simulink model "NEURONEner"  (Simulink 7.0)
settings: Solver=ode45  StartTime=0.0  StopTime=tstop  RelTol=1e-3
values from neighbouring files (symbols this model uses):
  beta = 1    [ResCourV1.m]    (also in ResCrV1.m; ResEnerV1.m; Constantes.m = 0.95; ConstantesBck.m = 0.95)
  Cdl = 731.3E-9    (= 7.313e-07)    [ResCourV1.m]    (also in ResCrV1.m; ResEnerV1.m; Constantes.m = 6.03e-07; ConstantesBck.m = 6.03e-07)
  I0Stim = ResSinhCorr(iRes,2)*1E-3    [ResCrV1.m]    (also in ResEnerV1.m; WaveCompIET.m = 0; WaveCompIETIf.m = 0)
  Rct = 605.2E3    (= 605200)    [ResCourV1.m]    (also in ResCrV1.m; ResEnerV1.m; Constantes.m = 185600; ConstantesBck.m = 185600)
  Rel = 2.09E3    (= 2090)    [ResCourV1.m]    (also in ResCrV1.m; ResEnerV1.m)
  sigma = 68000    [ResCourV1.m]    (also in ResCrV1.m; ResEnerV1.m; Constantes.m = 66466; ConstantesBck.m = 66466)
  T0Stim = ResSinhCorr(iRes,1)*1E-3    [ResCrV1.m]    (also in ResEnerV1.m; WaveCompIET.m = i; WaveCompIETIf.m = i)
  TypeStim = 11    [ResCrV1.m]    (also in ResEnerV1.m; WaveCompIET.m = 5; WaveCompIETIf.m = 5)
libraries: simulink x1

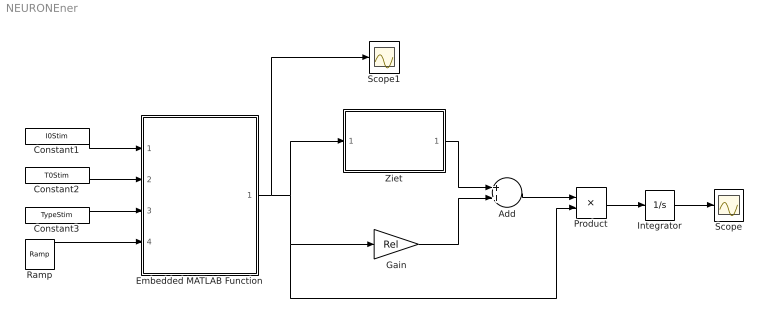
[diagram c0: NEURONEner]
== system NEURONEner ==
  Add : Sum  OutDataType=sfix(16)  OutScaling=2^-10
  Constant1 : Constant  Value=I0Stim  OutDataType=sfix(16)  OutScaling=2^0
  Constant2 : Constant  Value=T0Stim  OutDataType=sfix(16)  OutScaling=2^0
  Constant3 : Constant  Value=TypeStim  OutDataType=sfix(16)  OutScaling=2^0
  Embedded MATLAB Function : Stateflow chart
  Gain : Gain  Gain=Rel  ParameterDataType=sfix(16)  ParameterScaling=2^0  OutDataType=sfix(16)  OutScaling=2^0
  Integrator : Integrator
  Product : Product  OutDataType=sfix(16)  OutScaling=2^0
  Ramp : simulink/Sources/Ramp  SystemSampleTime=-1  slope=1  start=0  X0=0
  Scope : Scope
  Scope1 : Scope
  Ziet : Subsystem
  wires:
  Constant1/1 -> Embedded MATLAB Function/1(I0Stim)
  Constant2/1 -> Embedded MATLAB Function/2(T0Stim)
  Constant3/1 -> Embedded MATLAB Function/3(TypeStim)
  Ramp/1 -> Embedded MATLAB Function/4(temps)
  Embedded MATLAB Function/1(Istim) -> Ziet/1(InZiet), Gain/1, Product/2, Scope1/1
  Ziet/1(OutZiet) -> Add/1
  Gain/1 -> Add/2
  Product/1 -> Integrator/1
  Integrator/1 -> Scope/1
  Add/1 -> Product/1

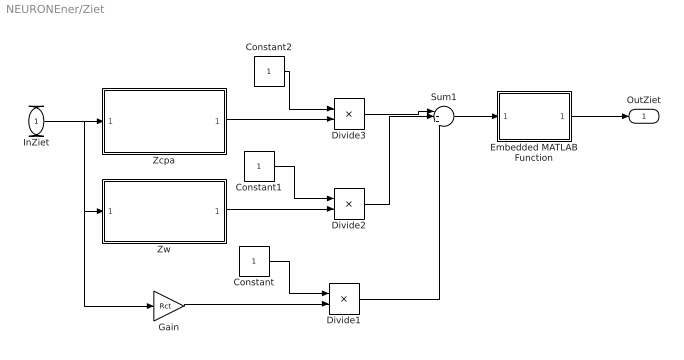
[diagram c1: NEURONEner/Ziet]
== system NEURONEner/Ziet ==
  InZiet : Inport  OutDataType=sfix(16)  OutScaling=2^0
  Constant : Constant  OutDataType=sfix(16)  OutScaling=2^0
  Constant1 : Constant  OutDataType=sfix(16)  OutScaling=2^0
  Constant2 : Constant  OutDataType=sfix(16)  OutScaling=2^0
  Divide1 : Product  Inputs=*/  OutDataType=sfix(16)  OutScaling=2^-10
  Divide2 : Product  Inputs=*/  OutDataType=sfix(16)  OutScaling=2^-10
  Divide3 : Product  Inputs=*/  OutDataType=sfix(16)  OutScaling=2^-10
  Embedded MATLAB Function : Stateflow chart
  Gain : Gain  Gain=Rct  ParameterDataType=sfix(16)  ParameterScaling=2^0  OutDataType=sfix(16)  OutScaling=2^0
  Sum1 : Sum  Inputs=|+++  OutDataType=sfix(16)  OutScaling=2^0
  Zcpa : Subsystem
  Zw : Subsystem
  OutZiet : Outport  OutDataType=sfix(16)  OutScaling=2^0
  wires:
  Constant/1 -> Divide1/1
  Constant1/1 -> Divide2/1
  Constant2/1 -> Divide3/1
  Zcpa/1(OutZcpa) -> Divide3/2
  Zw/1(OutZw) -> Divide2/2
  Sum1/1 -> Embedded MATLAB Function/1(u)
  Gain/1 -> Divide1/2
  InZiet/1 -> Zcpa/1(InZcpa), Zw/1(InZw), Gain/1
  Embedded MATLAB Function/1(y) -> OutZiet/1
  Divide1/1 -> Sum1/3
  Divide3/1 -> Sum1/1
  Divide2/1 -> Sum1/2

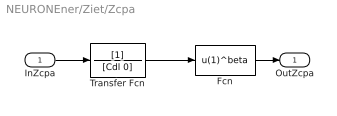
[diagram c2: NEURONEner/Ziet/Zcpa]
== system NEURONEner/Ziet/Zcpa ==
  InZcpa : Inport  OutDataType=sfix(16)  OutScaling=2^0
  Fcn : Fcn  Expr=u(1)^beta
  Transfer Fcn : TransferFcn  Denominator=[Cdl 0]
  OutZcpa : Outport  OutDataType=sfix(16)  OutScaling=2^0
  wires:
  Transfer Fcn/1 -> Fcn/1
  InZcpa/1 -> Transfer Fcn/1
  Fcn/1 -> OutZcpa/1

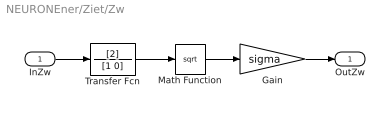
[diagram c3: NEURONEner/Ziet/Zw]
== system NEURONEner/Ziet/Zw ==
  InZw : Inport  OutDataType=sfix(16)  OutScaling=2^0
  Gain : Gain  Gain=sigma  ParameterDataType=sfix(16)  ParameterScaling=2^0  OutDataType=sfix(16)  OutScaling=2^0
  Math Function : Math  Operator=sqrt  OutDataType=sfix(16)  OutScaling=2^0
  Transfer Fcn : TransferFcn  Numerator=[2]  Denominator=[1 0]
  OutZw : Outport  OutDataType=sfix(16)  OutScaling=2^0
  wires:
  Transfer Fcn/1 -> Math Function/1
  Math Function/1 -> Gain/1
  Gain/1 -> OutZw/1
  InZw/1 -> Transfer Fcn/1

== matlab function Ziet/Embedded
MATLAB Function ==
function y = fcn(u)
% This block supports an embeddable subset of the MATLAB language.
% See the help menu for details. 

if u == Inf 
    y = 0;
else
    y = 1/u;
end

== matlab function Embedded
MATLAB Function ==
function Istim = courant(I0Stim,T0Stim,TypeStim,temps)
% This block supports an embeddable subset of the MATLAB language.
% See the help menu for details. 

if temps <= T0Stim
    if TypeStim == 0
        Iout = I0Stim;
    elseif TypeStim == 1
        Iout = I0Stim*sin(pi/T0Stim*temps);
    elseif TypeStim == 2
        Iout = I0Stim*sin(pi/(2*T0Stim)*temps);
    elseif TypeStim == 3
        taum=0.07492974E-3;
        Iout = I0Stim*exp(temps/taum);
    elseif TypeStim == 4
        taum=0.07492974E-3;
        Iout = I0Stim*exp(-temps/taum);
    elseif TypeStim == 5
        Iout = I0Stim*(sin(pi/T0Stim*temps)+1/3*sin(3*pi/T0Stim*temps));
    elseif TypeStim == 6   
        taum=0.07492974E-3;
        Iout = I0Stim*sinh(temps/taum);
    elseif TypeStim == 7
        Iout = I0Stim*temps;
    elseif TypeStim == 8
        Iout = I0Stim*(T0Stim-temps);
    elseif TypeStim == 9
        Iout = I0Stim*(exp(-(5/sqrt(2))*((temps-T0Stim/2)/T0Stim)^2));
    elseif TypeStim == 10
        taum=0.2008E-3;
        Iout = I0Stim*exp(temps/taum);
    else
        taum = 4.07749143E-3;
        Iout = I0Stim*sinh(temps/taum);        
    end
else
    Iout = 0;
end
Istim = Iout;
